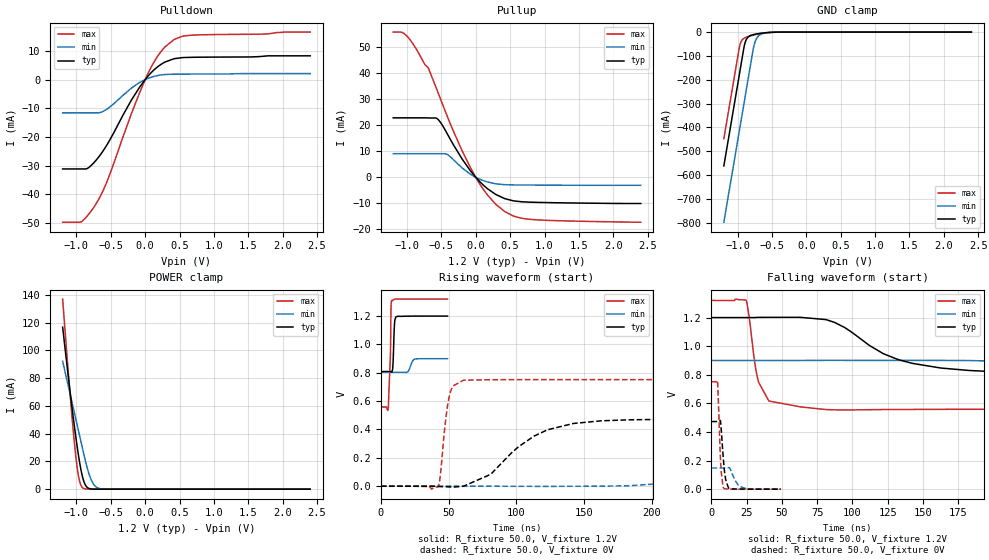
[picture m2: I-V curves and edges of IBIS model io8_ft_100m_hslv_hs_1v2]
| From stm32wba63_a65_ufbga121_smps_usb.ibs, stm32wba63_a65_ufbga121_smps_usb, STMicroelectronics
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[Model]   io8_ft_100m_hslv_hs_1v2
Model_type I/O
Polarity   Non-Inverting
Enable   Active-Low
| CAP_THRESHOLD on pad IOFT is "UDTCAPC" :
| Rising=30.0% of vddiom   Falling=70.0% of vddiom
| C_comp min and max val. don't necessarily correlate with the min and max pvt
| but are the smallest and greatest pad capacitance found.
| var   typ   min   max
C_comp   2.95990pF  2.88328pF  3.08656pF
|C_comp_pullup   1.71834pF  1.55891pF  1.87829pF
|C_comp_pulldown   1.24157pF  1.32437pF  1.20827pF
Vinl = 450.0mV
Vinh = 660.0mV
Vmeas = 600.0mV   | Reference voltage for timing measurements
Cref  = 50.0pF   | Timing specification test load capacitance value
Rref  = 1.0MOhm   | Timing specification test load resistance value
Vref  = 660.0mV   | Timing specification test load voltage
[Model Spec]
| TIME_THRESHOLD on pin ZIV11 is "CMOS" :
| Rising=50.0% of vdd   Falling=50.0% of vdd
Vinl 441.50000mV 335.50000mV 487.50000mV
Vinh 755.50000mV 552.50000mV 839.50000mV
| variable   typ   min   max
[Temperature Range] 25.0 140.0 -40.0
| variable   typ   min   max
[Voltage Range] 1.2V 900.0mV 1.32V
| variable   typ   min   max
[POWER Clamp Reference] 1.2V 900.0mV 1.32V
| variable   typ   min   max
[GND Clamp Reference] 0V 0V 0V
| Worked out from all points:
|   slope of the pulldown table from 0 to 0.18 V, typ, clamps not added: 40.6 ohm
|   slope of the pullup table from 0 to 0.18 V, typ, clamps not added: 39.6 ohm
|   GND clamp passes 1 mA (typ) near -0.51 V on its own axis
|   POWER clamp passes 1 mA (typ) near -0.83 V on its own axis
|   rising waveform, R_fixture 50.0, V_fixture 1.2V: 20-80 % time 851ps typ, 2.42ns min, 1.23ns max; typ from 0.809 V to 1.2 V
|   falling waveform, R_fixture 50.0, V_fixture 1.2V: 20-80 % time 43.8ns typ, 105ns min, 8.26ns max; typ from 1.2 V to 0.809 V
|   rising waveform, R_fixture 50.0, V_fixture 0V: 20-80 % time 36.5ns typ, 92.3ns min, 5.16ns max; typ from 0 V to 0.473 V
|   falling waveform, R_fixture 50.0, V_fixture 0V: 20-80 % time 2.46ns typ, 4.69ns min, 1.77ns max; typ from 0.473 V to 0 V
[POWER Clamp]
-1.2V     116.7mA    92.13mA    136.9mA
-1.09V    69.42mA    68.21mA    67.14mA
-1.02V    41.75mA    52.99mA    28.91mA
-990mV    30.98mA    46.47mA    16.09mA
-970mV    24.36mA    42.12mA    9.575mA
-940mV    15.59mA    35.6mA     3.485mA
-910mV    8.693mA    29.07mA    1.01mA
-860mV    2.259mA    18.59mA    104.6uA
-780mV    143.1uA    6.246mA    2.554uA
-720mV    16.22uA    1.846mA    157.1nA
-650mV    1.267uA    330.3uA    6.114nA
2.4V      0A         0A         0A
[GND Clamp]
-1.2V     -561.6mA   -797.4mA   -447.4mA
-980mV    -187.6mA   -423.4mA   -73.43mA
-960mV    -153.6mA   -389.4mA   -48.26mA
-900mV    -54.17mA   -287.4mA   -24.97mA
-870mV    -29.55mA   -236.4mA   -21.19mA
-830mV    -17.05mA   -168.4mA   -17.42mA
-760mV    -9.921mA   -54.55mA   -11.89mA
-730mV    -8.191mA   -29.78mA   -9.811mA
-690mV    -6.26mA    -14.49mA   -7.318mA
-600mV    -2.976mA   -4.315mA   -3.058mA
-380mV    -57.63uA   -251uA     -19.49uA
2.4V      871.4pA    205.6nA    347.3pA
| variable   typ   min   max
[Pullup Reference] 1.2V 900.0mV 1.32V
| variable   typ   min   max
[Pulldown Reference] 0V 0V 0V
[Pullup]
-1.2V     22.8mA     9.05mA     55.68mA
-1.06V    22.8mA     9.05mA     55.41mA
-950mV    22.8mA     9.05mA     52.53mA
-690mV    22.75mA    9.05mA     41.9mA
-560mV    22.44mA    9.05mA     33.24mA
-410mV    16.47mA    8.685mA    23.12mA
-200mV    7.069mA    3.642mA    10.26mA
0V        580.8fA    234pA      3fA
170mV     -4.361mA   -1.792mA   -6.756mA
420mV     -8.157mA   -2.82mA    -13.11mA
790mV     -9.528mA   -2.972mA   -16.12mA
2.4V      -10.04mA   -3.075mA   -17.21mA
[Pulldown]
-1.2V     -31.2mA    -11.62mA   -49.78mA
-930mV    -31.2mA    -11.62mA   -49.64mA
-830mV    -30.86mA   -11.62mA   -47.25mA
-710mV    -28.04mA   -11.62mA   -43.19mA
-550mV    -22.55mA   -10.2mA    -35.3mA
-200mV    -7.146mA   -2.964mA   -11.89mA
40mV      1.171mA    405.8uA    2.092mA
130mV     3.416mA    1.118mA    6.182mA
230mV     5.302mA    1.613mA    9.763mA
420mV     7.288mA    1.898mA    13.99mA
670mV     7.779mA    1.924mA    15.51mA
2.4V      8.3mA      2.094mA    16.59mA
[Ramp]
dV/dt_r 283.78486mV/7.20911ns 88.90733mV/18.32068ns 450.99611mV/1.03152ns
dV/dt_f 234.6597mV/8.69075ns 57.8937mV/20.71726ns 456.73566mV/1.48582ns
R_load = 50.0
| Removed startup time: 0s 0s 0s  .
| Removed end time: 49.25ns.
[Rising Waveform]
R_fixture   = 50.0
V_fixture   = 1.2V
V_fixture_min = 900.0mV
V_fixture_max = 1.32V
0s        808.9mV    803.5mV    558.8mV
5.45ns    808.9mV    803.5mV    555.3mV
7ns       808.9mV    803.5mV    913.3mV
7.45ns    808mV      803.5mV    1.233V
7.85ns    806.1mV    803.5mV    1.308V
8.7ns     825.7mV    803.5mV    1.308V
10.05ns   1.142V     803.5mV    1.319V
11.05ns   1.194V     803.5mV    1.32V
25.15ns   1.2V       897mV      1.32V
49.25ns   1.2V       899.7mV    1.32V
| Removed startup time: 0s 0s 0s  .
| Removed end time: 996.25ns.
[Falling Waveform]
R_fixture   = 50.0
V_fixture   = 1.2V
V_fixture_min = 900.0mV
V_fixture_max = 1.32V
0s        1.2V       900mV      1.32V
24.5ns    1.2V       900mV      1.321V
26.25ns   1.2V       900mV      1.237V
32.5ns    1.201V     900mV      786.1mV
40.75ns   1.202V     900mV      616.4mV
81.25ns   1.186V     900.7mV    556.8mV
132.3ns   907mV      900.5mV    557.2mV
203.3ns   820.5mV    894.8mV    558.7mV
386.5ns   809mV      813.1mV    558.8mV
996.2ns   808.9mV    803.5mV    558.8mV
| Removed startup time: 0s 0s 0s  .
| Removed end time: 996.25ns.
[Rising Waveform]
R_fixture   = 50.0
V_fixture   = 0V
V_fixture_min = 0V
V_fixture_max = 0V
0s        4.601nV    216.1nV    3.164nV
42.25ns   -1.282mV   918.1nV    -3.033mV
43.75ns   -2.25mV    912.1nV    61.55mV
50.75ns   -4.882mV   696.9nV    641.9mV
61ns      -361.7uV   113nV      747.4mV
81.25ns   84.24mV    21.1uV     751.4mV
113.3ns   353.8mV    -1.192mV   751.6mV
162.7ns   461.2mV    151uV      751.6mV
366ns     472.8mV    138.4mV    751.7mV
996.2ns   473mV      148.2mV    751.7mV
| Removed startup time: 0s 0s 0s  .
| Removed end time: 49.25ns.
[Falling Waveform]
R_fixture   = 50.0
V_fixture   = 0V
V_fixture_min = 0V
V_fixture_max = 0V
0s        473mV      148.3mV    751.7mV
4.3ns     473mV      148.3mV    754.3mV
6.6ns     459.4mV    148.3mV    170.7mV
7.1ns     393.6mV    148.3mV    107.4mV
8.5ns     204.3mV    148.3mV    9.317mV
10.05ns   68.91mV    148.2mV    2.564mV
12.5ns    4.653mV    151.7mV    887.8uV
18.1ns    765.1uV    40.48mV    185.4uV
21.15ns   423.5uV    15.06mV    92.42uV
49.25ns   5.633uV    152.4uV    46.05nV
